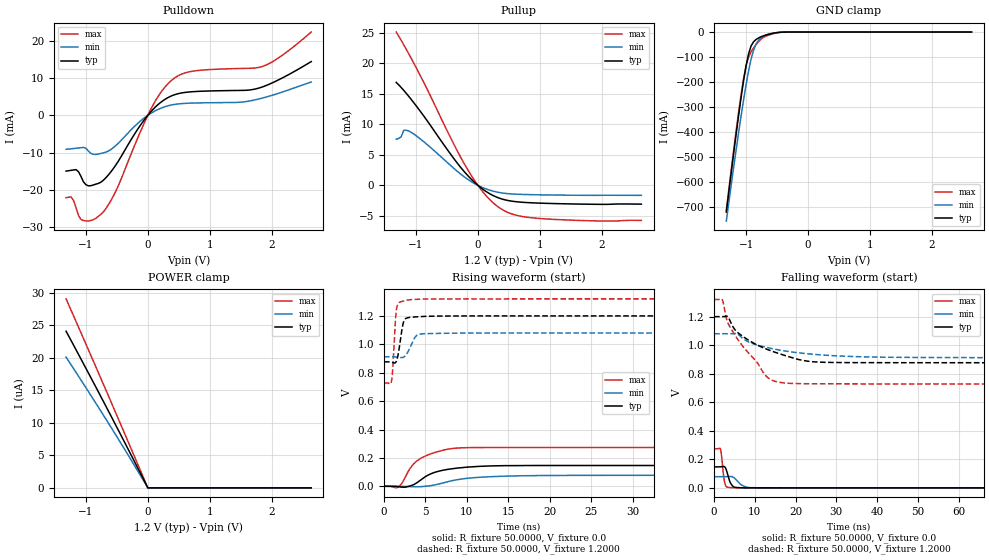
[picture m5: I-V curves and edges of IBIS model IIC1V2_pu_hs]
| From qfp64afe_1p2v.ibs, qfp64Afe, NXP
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[Model] IIC1V2_pu_hs
|   Model IIC1V2_pu_hs
| This model was characterised for following simulation conditions:
| External (pad) voltage:
|   - Typ: 1.2V,   - Min: 1.08V,   - Max: 1.32V
| Library cells for typ/min/max conditions are connected as defined below:
|  IO - External Pad
|  A - Core Input
|  EN - Output Buffer Enable
|  BOOST - vdde
|  EGP - vdd
|  EHS - vdd
|  ENZI - vdd
|  EPD - gnd
|  EPUN - gnd
|  ZI - NC
|  ZIF - NC
|  gnd - gnd
|  gnde - gnde
|  vdd - vdd
|  vdde - vdde
| All other pins connected to ground
Model_type I/O
Polarity   Non-Inverting
Enable   Active-Low
Vinl =   0.5400V
Vinh =   1.2600V
Vmeas =  0.9000V
Cref =   0.0F
Rref =   1.0000k
Vref =   0.0V
C_comp   3.6132pF   3.4729pF   3.7394pF
|C_comp_pullup   0.9305pF   0.8897pF   0.9448pF
|C_comp_pulldown   2.3306pF   2.4843pF   2.1848pF
[Model Spec]
| variable   typ   min   max
Vinh   0.3600V   0.3240V   0.3960V
Vinl   0.8400V   0.7560V   0.9240V
Vmeas   0.6000V   0.5400V   0.6600V
[Temperature Range]   25.0000   0.1250k   -40.0000
[Voltage Range]   1.2000V   1.0800V   1.3200V
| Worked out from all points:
|   slope of the pulldown table from 0 to 0.18 V, typ, clamps not added: 58.3 ohm
|   slope of the pullup table from 0 to 0.18 V, typ, clamps not added: 138 ohm
|   GND clamp passes 1 mA (typ) near -0.45 V on its own axis
|   rising waveform, R_fixture 50.0000, V_fixture 0.0: 20-80 % time 3.44ns typ, 4.6ns min, 2.72ns max; typ from 0.001 V to 0.147 V
|   rising waveform, R_fixture 50.0000, V_fixture 1.2000: 20-80 % time 518ps typ, 829ps min, 343ps max; typ from 0.877 V to 1.2 V
|   falling waveform, R_fixture 50.0000, V_fixture 0.0: 20-80 % time 1.03ns typ, 1.79ns min, 625ps max; typ from 0.147 V to 0.001 V
|   falling waveform, R_fixture 50.0000, V_fixture 1.2000: 20-80 % time 11.4ns typ, 13.9ns min, 8.37ns max; typ from 1.2 V to 0.877 V
[Pulldown]
|Voltage   I(typ)   I(min)   I(max)
-1.32V    -14.96mA   -9.099mA   -22.09mA
-1.24V    -14.75mA   -8.982mA   -21.89mA
-1.16V    -14.56mA   -8.83mA    -24.7mA
-1.04V    -17.82mA   -8.609mA   -28.21mA
-920mV    -18.88mA   -10.21mA   -28.21mA
-720mV    -17.44mA   -10.07mA   -25.94mA
-520mV    -13.41mA   -8.157mA   -20.44mA
80mV      1.521mA    840uA      2.628mA
440mV     5.569mA    2.951mA    10.1mA
760mV     6.377mA    3.307mA    11.92mA
1.84V     7.555mA    4.581mA    13.06mA
2.64V     14.41mA    8.944mA    22.34mA
[Pullup]
|Voltage   I(typ)   I(min)   I(max)
-1.32V    16.86mA    7.552mA    25.1mA
-1.24V    16.02mA    7.934mA    23.74mA
-1.2V     15.57mA    8.992mA    23.04mA
-1.08V    14.09mA    8.685mA    20.84mA
-400mV    4.539mA    2.883mA    6.954mA
-200mV    2.009mA    1.241mA    3.176mA
80mV      -640.3uA   -373.7uA   -1.07mA
320mV     -1.996mA   -1.123mA   -3.467mA
560mV     -2.602mA   -1.412mA   -4.719mA
920mV     -2.876mA   -1.532mA   -5.352mA
1.96V     -3.103mA   -1.628mA   -5.823mA
2.64V     -3.069mA   -1.636mA   -5.736mA
[GND_clamp]
|Voltage   I(typ)   I(min)   I(max)
-1.32V    -720.7mA   -756.5mA   -713.8mA
-1.12V    -330.9mA   -399.5mA   -316.8mA
-1.04V    -192.5mA   -269.2mA   -184.5mA
-1V       -133.6mA   -209.3mA   -133.5mA
-960mV    -86.76mA   -154.8mA   -99.49mA
-920mV    -55.71mA   -108.2mA   -79.05mA
-880mV    -39.04mA   -72.36mA   -63.74mA
-840mV    -29.93mA   -48.01mA   -50.29mA
-760mV    -18.95mA   -23.41mA   -28.35mA
-640mV    -9.243mA   -8.645mA   -12.76mA
-400mV    -357.8uA   -419.3uA   -472.1uA
2.64V     0A         0A         0A
[POWER_clamp]
|Voltage   I(typ)   I(min)   I(max)
-1.32V    24.09uA    20.1uA     29.06uA
-640mV    11.88uA    10.01uA    14.23uA
0V        86.89pA    4.342nA    7.851pA
2.64V     0A         0A         0A
[Ramp]
| variable   typ   min   max
dV/dt_r  88.0047m/3.4385n   46.5618m/4.5994n   0.1640/2.7251n
dV/dt_f  0.1939/11.3745n   0.1006/13.8670n   0.3549/8.3686n
R_load = 50.0000
[Rising Waveform]
R_fixture= 50.0000
V_fixture= 0.0
V_fixture_min= 0.0
V_fixture_max= 0.0
|time   V(typ)   V(min)   V(max)
0s        557uV      548.4uV    536.1uV
1.691ns   -1.647mV   716.1uV    -5.154mV
2.17ns    -5.445mV   576.4uV    22.31mV
3.014ns   518uV      -1.73mV    113.9mV
3.549ns   11.25mV    -3.106mV   156.3mV
5.337ns   79.59mV    3.025mV    222.2mV
8.063ns   122.9mV    38.08mV    265.3mV
11.59ns   141.1mV    64.25mV    273.5mV
33.29ns   147.2mV    77.97mV    273.9mV
1us       147.2mV    78.15mV    273.9mV
[Rising Waveform]
R_fixture= 50.0000
V_fixture= 1.2000
V_fixture_min= 1.0800
V_fixture_max= 1.3200
|time   V(typ)   V(min)   V(max)
0s        876.9mV    912.3mV    728.5mV
905.7ps   874.4mV    912.7mV    738.3mV
1.071ns   871.2mV    912.5mV    835mV
1.419ns   872.7mV    910.8mV    1.197V
1.687ns   920.5mV    908.9mV    1.283V
2.226ns   1.122V     907mV      1.303V
2.558ns   1.179V     917.7mV    1.308V
3.966ns   1.194V     1.064V     1.317V
5.905ns   1.198V     1.076V     1.319V
1us       1.2V       1.08V      1.32V
[Falling Waveform]
R_fixture= 50.0000
V_fixture= 0.0
V_fixture_min= 0.0
V_fixture_max= 0.0
|time   V(typ)   V(min)   V(max)
0s        147.2mV    78.15mV    273.9mV
1.585ns   147.6mV    78.14mV    270.1mV
1.819ns   148.6mV    78.11mV    229.2mV
2.381ns   150.6mV    78.11mV    74.02mV
2.874ns   135.7mV    78.75mV    13.18mV
4.167ns   28.04mV    79.95mV    2.051mV
5.762ns   2.352mV    46.37mV    878.5uV
8.091ns   857.1uV    4.716mV    598.7uV
13.79ns   576.6uV    656.2uV    541uV
1us       557uV      548.4uV    536.1uV
[Falling Waveform]
R_fixture= 50.0000
V_fixture= 1.2000
V_fixture_min= 1.0800
V_fixture_max= 1.3200
|time   V(typ)   V(min)   V(max)
0s        1.2V       1.08V      1.32V
1.972ns   1.2V       1.08V      1.323V
3.033ns   1.203V     1.08V      1.186V
3.957ns   1.168V     1.08V      1.125V
6.24ns    1.079V     1.067V     1.023V
12.94ns   971.6mV    984.3mV    778.9mV
20.09ns   904.8mV    948.7mV    731.1mV
27.28ns   879.9mV    929.9mV    729.2mV
63.74ns   877.1mV    913mV      728.6mV
1us       876.9mV    912.3mV    728.5mV
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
